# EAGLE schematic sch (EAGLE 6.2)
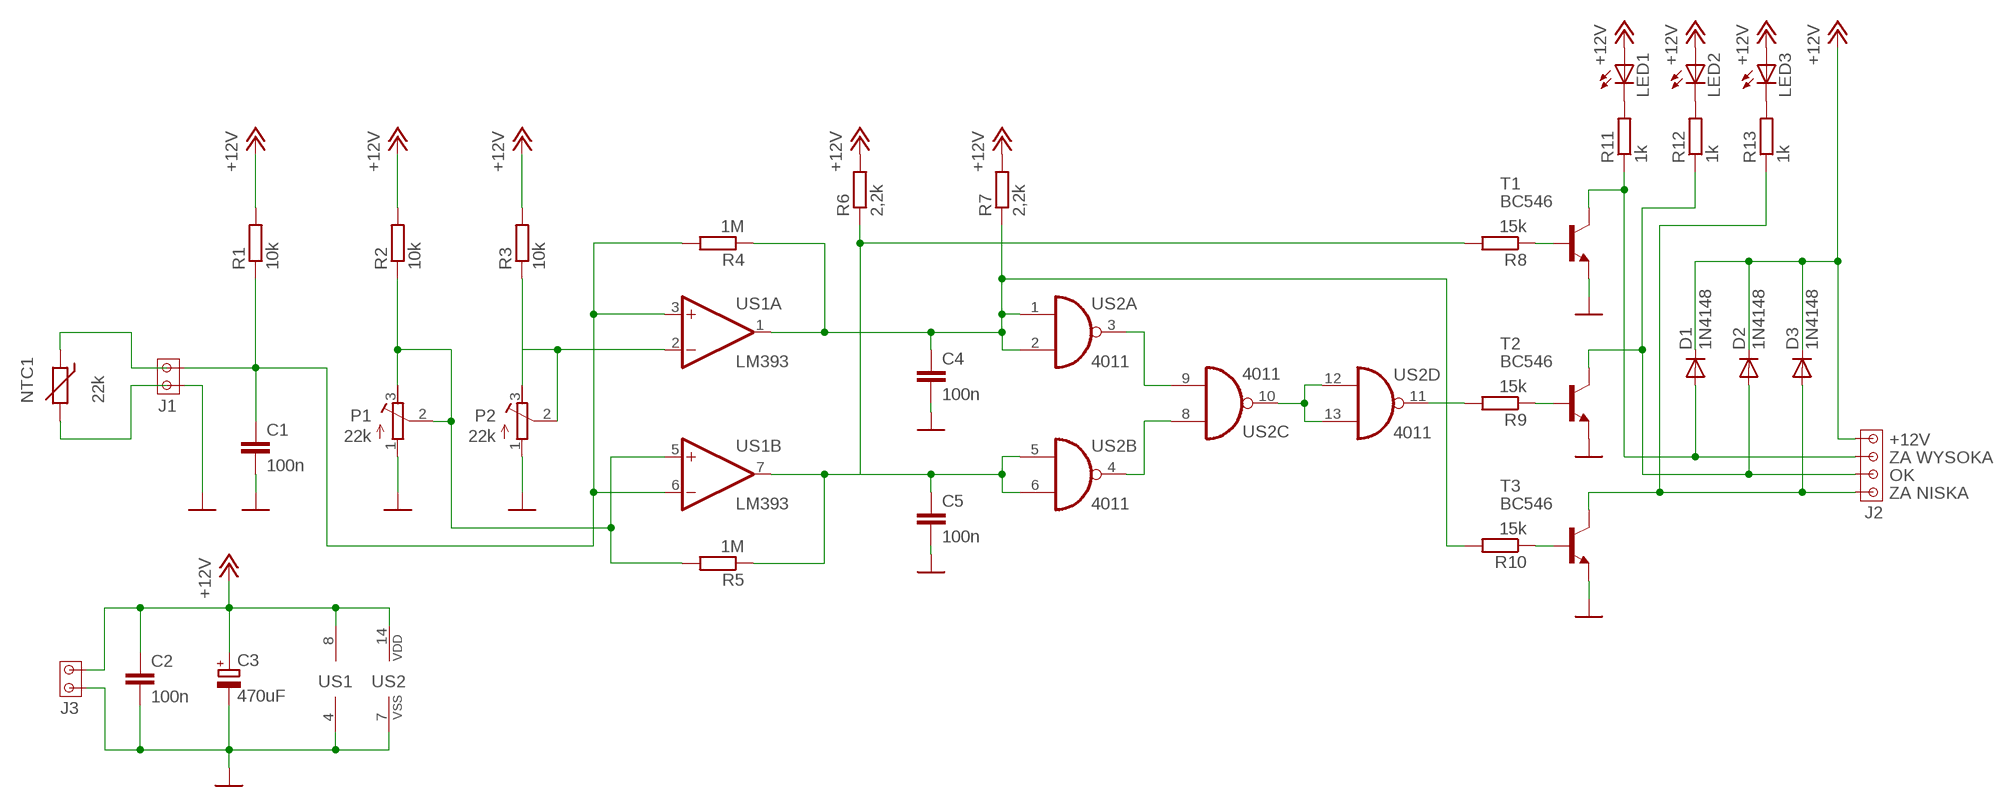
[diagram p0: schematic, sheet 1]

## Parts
C1  100n  C-EU025-024X044  [C025-024X044]
C2  100n  C-EU025-024X044  [C025-024X044]
C3  470uF  CPOL-EU085CS-1AR  [085CS_1AR]
C4  100n  C-EU025-024X044  [C025-024X044]
C5  100n  C-EU025-024X044  [C025-024X044]
D1  1N4148  1N4148DO35-10  [DO35-10]
D2  1N4148  1N4148DO35-10  [DO35-10]
D3  1N4148  1N4148DO35-10  [DO35-10]
LED1  LED5MM  [LED5MM]
LED2  LED5MM  [LED5MM]
LED3  LED5MM  [LED5MM]
NTC1  22k  THERMISTOR-7,5  [R-7,5]
P1  22k  R-TRIMM4G/J  [RTRIM4G/J]
P2  22k  R-TRIMM4G/J  [RTRIM4G/J]
R1  10k  R-EU_0204/2V  [0204V]
R2  10k  R-EU_0204/2V  [0204V]
R3  10k  R-EU_0204/2V  [0204V]
R4  1M  R-EU_0204/2V  [0204V]
R5  1M  R-EU_0204/2V  [0204V]
R6  2,2k  R-EU_0204/2V  [0204V]
R7  2,2k  R-EU_0204/2V  [0204V]
R8  15k  R-EU_0204/2V  [0204V]
R9  15k  R-EU_0204/2V  [0204V]
R10  15k  R-EU_0204/2V  [0204V]
R11  1k  R-EU_0204/2V  [0204V]
R12  1k  R-EU_0204/2V  [0204V]
R13  1k  R-EU_0204/2V  [0204V]
T1  BC546  2N706  [TO18]
T2  BC546  2N706  [TO18]
T3  BC546  2N706  [TO18]
US1  LM393  LM393N  [DIL08]
US2  4011  4011N  [DIL14]

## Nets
+12V: C2.1 C3.+ D1.C D2.C D3.C LED1.A LED2.A LED3.A R1.2 R2.2 R3.2 R6.2 R7.2 US1.8(P:V+) US2.14(P:VDD)
GND: C1.2 C2.2 C3.- C4.2 C5.2 P1.1(E) P2.1(E) T1.1(E) T2.1(E) T3.1(E) US1.4(P:V-) US2.7(P:VSS)
N$1: NTC1.2
N$2: NTC1.1
N$3: C1.1 R1.1 R4.2 US1.3(A:+IN) US1.6(B:-IN)
N$4: P1.2(S) P1.3(A) R2.1 R5.2 US1.5(B:+IN)
N$5: C5.1 R5.1 R6.1 R8.2 US1.7(B:OUT) US2.5(B:I0) US2.6(B:I1)
N$6: P2.2(S) P2.3(A) R3.1 US1.2(A:-IN)
N$7: C4.1 R4.1 R7.1 R10.2 US1.1(A:OUT) US2.1(A:I0) US2.2(A:I1)
N$8: D1.A R11.1 T1.3(C)
N$9: D2.A R12.1 T2.3(C)
N$10: US2.4(B:O) US2.8(C:I0)
N$11: US2.3(A:O) US2.9(C:I1)
N$12: US2.10(C:O) US2.12(D:I0) US2.13(D:I1)
N$13: R9.2 US2.11(D:O)
N$14: D3.A R13.1 T3.3(C)
N$15: R10.1 T3.2(B)
N$16: R9.1 T2.2(B)
N$17: R8.1 T1.2(B)
N$18: LED1.K(C) R11.2
N$19: LED2.K(C) R12.2
N$20: LED3.K(C) R13.2

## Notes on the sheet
- J1
- +12V
- ZA WYSOKA
- OK
- ZA NISKA
- J2
- US1 | US2
- J3

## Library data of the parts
C1 C2 C4 C5 = rcl:C-EU: CAPACITOR, European symbol
C3 = rcl:CPOL-EU: POLARIZED CAPACITOR, European symbol
D1-D3 = diode:1N4148: DIODE
LED1-LED3 = led:LED: LED
NTC1 = varistor:THERMISTOR: THERMISTOR
P1 P2 = rcl:R-TRIMM: Trimm resistor
R1-R13 = rcl:R-EU_: RESISTOR, European symbol
T1-T3 = transistor-npn:2N706: NPN Transistor
US1 = linear:LM393: COMPARATOR
US2 = 40xx:4011: Quad 2-input NAND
